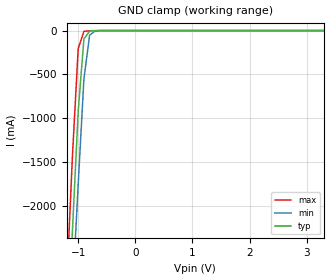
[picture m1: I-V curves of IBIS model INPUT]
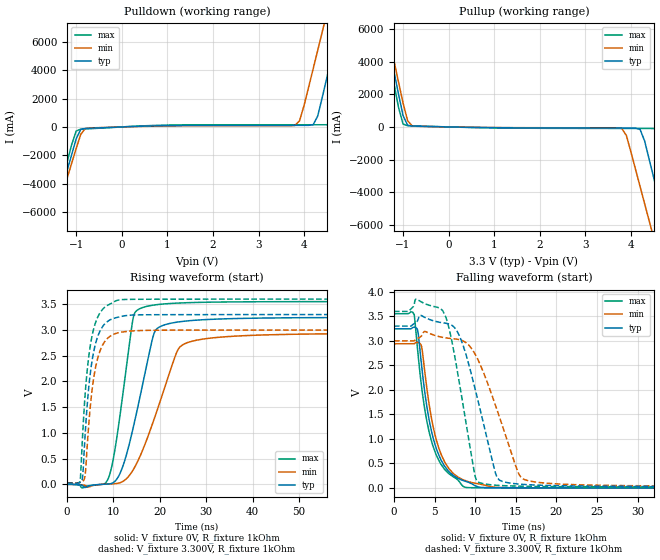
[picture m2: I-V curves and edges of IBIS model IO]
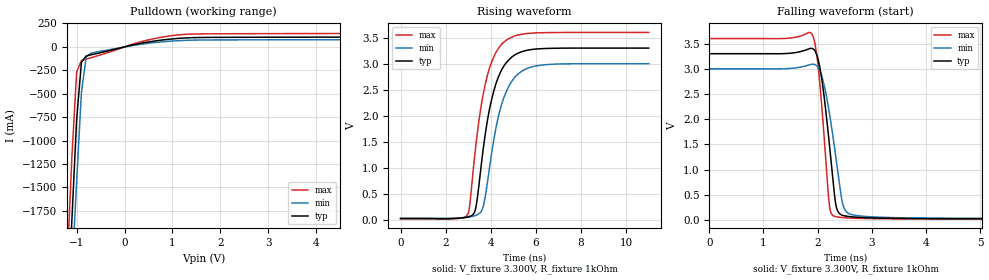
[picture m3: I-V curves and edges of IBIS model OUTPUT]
|   PERICOM SEMICONDUCTOR CORP
|   IBIS Model of PI4IOE5V9554
|   Product Family: 4IOE
|   16-TSSOP Package (L)
[IBIS Ver] 3.2
[Comment char] |_char
[File Name] pi4ioe5v9554_l_33v.ibs
[File ReV] 1.0
[Source] File originated at Pericom Semiconductor Corp.
[Date] 12/31/15
[Disclaimer] (C) Copyright PERICOM Semiconductor Corporation
   All rights reserved
  Pericom Semiconductor Corporation hereby grants the user of
  this IBIS model a non-exclusive, nontransferable license to
  use this IBIS model under the following terms.
  This IBIS model is provided on an "AS IS" basis and Pericom
  makes absolutely no warranty with respect to the information
  contained herein. PERICOM DISCLAIMS AND CUSTOMER WAIVES ALL
  WARRANTIES, EXPRESSED OR IMPLIED, INCLUDING WARRANTIES OF
  MERCHANTABILITY OR FITNESS FOR A PARTICULAR PURPOSE. The
  entire risk as to quality and performance is with the customer.
  Accordingly, in no event shall the company be liable for any
  damages, whether in contract or tort, including any lost
  profits or other incidental, consequential, exemplary, or
  punitive damages arising out of the use or application of the
  IBIS model provided in this package. Further, Pericom reserves
  the right to make changes without notice to any product herein
  to improve reliability, function, or design. Pericom does not
  convey any license under patent rights or any other intellectual
  property rights, including those of third parties.
  The user is granted this license only to use the IBIS model
  and is not granted rights to sell, load, rent, lease or license
  the IBIS model in whole or in part, or in modified form to anyone
  other than user. User may modify the IBIS model to suit its specific
  application but rights to derivative works and such modifications
  shall belong to Pericom.
  Pericom is not obligated to provide maintenance or support
  for the licensed IBIS model.
  Contact Pericom at ATTN: APPLICATION ENGINEERING / IBIS MODELS
  1545 Barber Lane Milpitas, CA 95035 USA.
[Component] PI4IOE5V9554
[Manufacturer] Pericom Semiconductor Corp.
[Package]
| Variable   typ   min   max
R_pkg   0.07795ohm   0.06700ohm   0.08890ohm
L_pkg   2.39150nH   2.22200nH   2.56100nH
C_pkg   0.38400pF   0.31500pF   0.45300pF
[Pin]  signal_name   model_name   R_pin   L_pin   C_pin
1   A0   INPUT   0.08890   2.56100nH   0.45300pF
2   A1   INPUT   0.08160   2.44800nH   0.40700pF
3   A2   INPUT   0.07430   2.33500nH   0.36100pF
4   IO0   IO   0.06700   2.22200nH   0.31500pF
5   IO1   IO   0.06700   2.22200nH   0.31500pF
6   IO2   IO   0.07430   2.33500nH   0.36100pF
7   IO3   IO   0.08160   2.44800nH   0.40700pF
8   GND   GND   0.08890   2.56100nH   0.45300pF
9   IO4   IO   0.08890   2.56100nH   0.45300pF
10   IO5   IO   0.08160   2.44800nH   0.40700pF
11   IO6   IO   0.07430   2.33500nH   0.36100pF
12   IO7   IO   0.06700   2.22200nH   0.31500pF
13   _INT   OUTPUT   0.06700   2.22200nH   0.31500pF
14   SCL   INPUT   0.07430   2.33500nH   0.36100pF
15   SDA   IO_OD   0.08160   2.44800nH   0.40700pF
16   VCC   POWER   0.08890   2.56100nH   0.45300pF
| Models and submodels in the file (4): INPUT (Input), IO (I/O), OUTPUT (Open_drain), IO_OD (I/O_open_drain)
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|   Model INPUT
[Model] INPUT
Model_type Input
Vinl = 800mV
Vinh = 2.00V
| Variable   typ   min   max
C_comp   3.700p   3.650p   3.750p
[Voltage Range]   3.300V   3.000V   3.600V
[POWER Clamp Reference]   3.300V   3.000V   3.600V
[GND Clamp Reference]   0.000V   0.000V   0.000V
[temperature range]   25   85   -40
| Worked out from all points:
|   GND clamp passes 1 mA (typ) near -0.67 V on its own axis
[GND Clamp]
| Voltage   I(typ)   I(min)   I(max)
-3.3V     -31.95A    -30.77A    -33.53A
-1.2V     -3.619A    -4.277A    -2.881A
-1.1V     -2.269A    -3.016A    -1.422A
-1V       -921.7mA   -1.755A    -206mA
-900mV    -95.47mA   -552.8mA   -8.619mA
-800mV    -5.698mA   -51.42mA   -2.791mA
-700mV    -1.267mA   -3.839mA   -635.9uA
3.3V      81.1pA     220.5pA    79.2pA
[POWER Clamp]
| Voltage   I(typ)   I(min)   I(max)
-3.3V     0A         0A         0A
3.3V      0A         0A         0A
|   Model IO
[Model]   IO
Model_type  I/O
Vinl = 800mV
Vinh = 2.00V
Vref =  0V
Vmeas = 0V
| Variable   typ   min   max
C_comp   3.700p   3.650p   3.750p
[Voltage Range]   3.300V   3.000V   3.600V
[Temperature Range]   25   85   -40
[Pullup Reference]   3.300V   3.000V   3.600V
[Pulldown Reference]   0.000V   0.000V   0.000V
[POWER Clamp Reference]   3.300V   3.000V   3.600V
[GND Clamp Reference]   0.000V   0.000V   0.000V
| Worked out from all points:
|   slope of the pulldown table from 0 to 0.495 V, typ, clamps not added: 8.87 ohm
|   slope of the pullup table from 0 to 0.495 V, typ, clamps not added: 18.9 ohm
|   falling waveform, V_fixture 0V, R_fixture 1kOhm: 20-80 % time 2.24ns typ, 2.27ns min, 2.22ns max; typ from 3.25 V to 0 V
|   rising waveform, V_fixture 0V, R_fixture 1kOhm: 20-80 % time 4.81ns typ, 6.84ns min, 3.22ns max; typ from 0 V to 3.25 V
|   falling waveform, V_fixture 3.300V, R_fixture 1kOhm: 20-80 % time 2.93ns typ, 3.74ns min, 2.21ns max; typ from 3.3 V to 0.025 V
|   rising waveform, V_fixture 3.300V, R_fixture 1kOhm: 20-80 % time 2.19ns typ, 2.22ns min, 2.16ns max; typ from 0.024 V to 3.3 V
[GND Clamp]
| Voltage   I(typ)   I(min)   I(max)
-3.3V     0A         0A         0A
3.3V      0A         0A         0A
[POWER Clamp]
| Voltage   I(typ)   I(min)   I(max)
-3.3V     0A         0A         0A
3.3V      0A         0A         0A
[Pulldown]
| Voltage   I(typ)   I(min)   I(max)
-3.3V     -26.81A    -25.73A    -28.23A
-1.6V     -7.608A    -7.837A    -7.392A
-1.1V     -1.96A     -2.573A    -1.261A
-900mV    -175.7mA   -518.3mA   -155.7mA
3.8V      111.2mA    106.5mA    152.4mA
3.9V      111.3mA    429.6mA    152.5mA
4.2V      158.7mA    4.111A     152.8mA
4.4V      2.103A     6.724A     153.4mA
4.6V      4.861A     9.342A     268mA
4.8V      7.635A     11.96A     2.796A
5.1V      11.8A      15.89A     7.245A
6.6V      32.65A     35.55A     29.58A
[Pullup]
| Voltage   I(typ)   I(min)   I(max)
-3.3V     32.55A     31.55A     33.88A
-1.4V     6.157A     6.662A     5.629A
-1.1V     2.012A     2.748A     1.196A
-900mV    100.8mA    378.4mA    74.56mA
3.8V      -68.24mA   -97.16mA   -90.16mA
4.2V      -150.7mA   -3.643A    -90.92mA
4.4V      -1.987A    -5.747A    -93.63mA
4.5V      -3.116A    -6.799A    -98.83mA
4.6V      -4.245A    -7.851A    -268.1mA
4.8V      -6.502A    -9.956A    -2.528A
5.1V      -9.888A    -13.11A    -6.204A
6.6V      -26.82A    -28.9A     -24.59A
[Falling Waveform]
V_fixture = 0V
V_fixture_min = 0V
V_fixture_max = 0V
R_fixture = 1kOhm
C_fixture = 0F
|   Time   V(typ)   V(min)   V(max)
0s        3.245V     2.939V     3.553V
2.5ns     3.281V     2.942V     3.534V
2.9ns     3.228V     2.971V     2.843V
3.3ns     2.662V     2.926V     2.206V
4.3ns     1.419V     1.741V     1.166V
5.5ns     683.3mV    824mV      570.6mV
6.8ns     327.6mV    385.9mV    286.2mV
8.7ns     140.2mV    153.9mV    14.36mV
13.2ns    2.566mV    7.029mV    1.232mV
50ns      282.3uV    397uV      193.3uV
[Rising Waveform]
V_fixture = 0V
V_fixture_min = 0V
V_fixture_max = 0V
R_fixture = 1kOhm
C_fixture = 0F
|   Time   V(typ)   V(min)   V(max)
0s        237.8uV    294uV      180.5uV
8.8ns     5.961mV    7.334mV    96.59mV
10ns      37.28mV    11.47mV    513.5mV
11.4ns    210mV      30.91mV    1.336V
14.2ns    1.081V     274.1mV    3.214V
16.1ns    1.863V     623.9mV    3.43V
19.1ns    3V         1.357V     3.49V
23.6ns    3.152V     2.559V     3.522V
26ns      3.178V     2.757V     3.531V
100ns     3.245V     2.939V     3.553V
[Falling Waveform]
V_fixture = 3.300V
V_fixture_min = 3.000V
V_fixture_max = 3.600V
R_fixture = 1kOhm
C_fixture = 0F
|   Time   V(typ)   V(min)   V(max)
0s        3.3V       3V         3.6V
2.7ns     3.372V     3.029V     3.851V
6ns       3.367V     3.071V     3.618V
6.88ns    3.338V     3.05V      3.19V
8.08ns    3.098V     3.022V     2.12V
9.88ns    2.095V     2.761V     335.5mV
10.36ns   1.774V     2.61V      120.5mV
12.7ns    213.3mV    1.589V     52.51mV
16ns      70.07mV    174.1mV    33.14mV
50ns      24.96mV    32.07mV    18.55mV
[Rising Waveform]
V_fixture = 3.300V
V_fixture_min = 3.000V
V_fixture_max = 3.600V
R_fixture = 1kOhm
C_fixture = 0F
|   Time   V(typ)   V(min)   V(max)
0s        24.32mV    30.04mV    18.43mV
2.8ns     38.19mV    36.5mV     71.73mV
3.4ns     188.4mV    62.07mV    1.039V
3.9ns     972.5mV    178.2mV    1.757V
4.7ns     1.912V     1.194V     2.501V
5.7ns     2.562V     2.044V     3.009V
6.6ns     2.872V     2.451V     3.25V
7.6ns     3.058V     2.697V     3.396V
10.4ns    3.235V     2.929V     3.562V
100ns     3.3V       3V         3.6V
[Ramp]
| Variable   typ   min   max
dV/dt_r   1.94712V/4.7977n   1.76334V/6.8391n   2.13138V/3.2275n
dV/dt_f   1.78188V/3.7400n   1.96536V/2.9308n   2.14896V/2.2014n
R_load = 1000
|   Model OUTPUT
[Model]   OUTPUT
Model_type  Open_drain
Vref =  3.300V
Rref =  1k
Cref =  0
Vmeas = 1.650V
| Variable   typ   min   max
C_comp   4.000p   3.950p   4.050p
[Voltage Range]   3.300V   3.000V   3.600V
[Temperature Range]   25   85   -40
[Pullup Reference]   3.300V   3.000V   3.600V
[Pulldown Reference]   0.000V   0.000V   0.000V
[POWER Clamp Reference]   3.300V   3.000V   3.600V
[GND Clamp Reference]   0.000V   0.000V   0.000V
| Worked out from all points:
|   slope of the pulldown table from 0 to 0.495 V, typ, clamps not added: 9.5 ohm
|   falling waveform, V_fixture 3.300V, R_fixture 1kOhm: 20-80 % time 198ps typ, 244ps min, 157ps max; typ from 3.3 V to 0.026 V
|   rising waveform, V_fixture 3.300V, R_fixture 1kOhm: 20-80 % time 775ps typ, 812ps min, 748ps max; typ from 0.026 V to 3.3 V
[GND Clamp]
| Voltage   I(typ)   I(min)   I(max)
-3.3V     0A         0A         0A
3.3V      0A         0A         0A
[POWER Clamp]
| Voltage   I(typ)   I(min)   I(max)
-3.3V     0A         0A         0A
3.3V      0A         0A         0A
[Pulldown]
| Voltage   I(typ)   I(min)   I(max)
-3.3V     -25.6A     -24.64A    -26.87A
-1.2V     -2.931A    -3.451A    -2.349A
-1.1V     -1.851A    -2.442A    -1.181A
-1V       -776.1mA   -1.433A    -269.4mA
-900mV    -163.2mA   -482.5mA   -144.6mA
-800mV    -96.66mA   -106.4mA   -129.8mA
-700mV    -84.43mA   -66.21mA   -115.6mA
400mV     43.75mA    32.2mA     62.54mA
800mV     74.26mA    54.46mA    105.7mA
1.2V      93.45mA    68.16mA    131.7mA
5.3V      107mA      78.44mA    147.2mA
6.6V      128mA      93.61mA    179.1mA
[Falling Waveform]
V_fixture = 3.300V
V_fixture_min = 3.000V
V_fixture_max = 3.600V
R_fixture = 1kOhm
C_fixture = 0F
|   Time   V(typ)   V(min)   V(max)
0s        3.3V       3V         3.6V
1.9ns     3.404V     3.091V     3.682V
2ns       3.227V     3.043V     3.146V
2.08ns    2.776V     2.85V      2.219V
2.21ns    1.583V     2.172V     358.8mV
2.3ns     624.3mV    1.534V     79.52mV
2.365ns   193.4mV    1.027V     61.54mV
2.47ns    90.84mV    293.2mV    48.44mV
2.65ns    62.33mV    102.6mV    36.9mV
8ns       25.8mV     31.84mV    19.55mV
[Rising Waveform]
V_fixture = 3.300V
V_fixture_min = 3.000V
V_fixture_max = 3.600V
R_fixture = 1kOhm
C_fixture = 0F
|   Time   V(typ)   V(min)   V(max)
0s        25.8mV     31.83mV    19.55mV
3ns       57.76mV    53.57mV    123.6mV
3.33ns    225.1mV    85.7mV     1.402V
3.6ns     1.14V      180.9mV    2.261V
3.75ns    1.635V     441.9mV    2.6V
4.22ns    2.605V     1.749V     3.21V
4.62ns    2.981V     2.397V     3.43V
5.22ns    3.205V     2.807V     3.553V
5.94ns    3.279V     2.952V     3.591V
11ns      3.3V       3V         3.6V
[Ramp]
| Variable   typ   min   max
dV/dt_r   1.96452V/770.74p   1.78092V/808.51p   2.14830V/748.57p
dV/dt_f   1.96452V/198.04p   1.78092V/243.82p   2.14830V/155.87p
R_load = 1000
